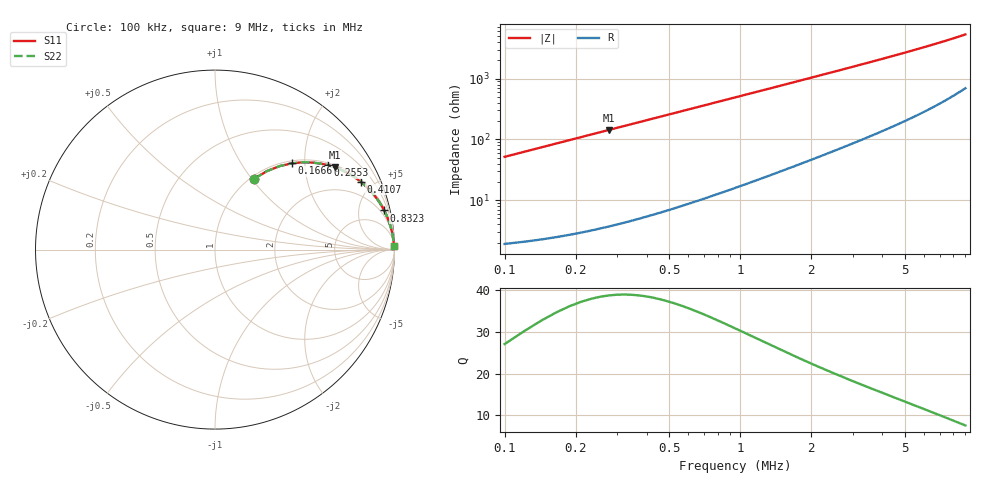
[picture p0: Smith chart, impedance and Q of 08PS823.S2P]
! Coilcraft 0805PS-823 Power Chip Inductor
! 5 February 2003
# MHZ S MA R 50
!Freq  MagS11  AngS11  MagS21  AngS21  MagS12  AngS12  MagS22  AngS22
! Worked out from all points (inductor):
!   403 points, 100 kHz to 9 MHz, reference 50 ohm
!   read as one part in series: L = 82 uH near 144.4 kHz
!   highest Q = 38.8 at 277.5 kHz (marker M1), where L = 82 uH
!   S11 on the Smith chart (normalised r, x): 100 kHz: 1.04, +1.03; 166.6 kHz: 1.05, +1.72; 255.3 kHz: 1.07, +2.63; 410.7 kHz: 1.11, +4.23; 832.3 kHz: 1.26, +8.58; 9 MHz: open
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0.1  0.4515 61.1  0.8758 -26.8  0.8758 -26.8  0.4515 61.1
0.12219  0.5252 56.5  0.8339 -31.7  0.8339 -31.7  0.5252 56.5
0.16657  0.6423 48.4  0.7482 -39.9  0.7482 -39.9  0.6423 48.4
0.21095  0.7263 41.9  0.6681 -46.6  0.6681 -46.6  0.7263 41.9
0.25533  0.7864 36.7  0.5977 -51.8  0.5977 -51.8  0.7864 36.7
0.27752  0.8098 34.5  0.5662 -54.0  0.5662 -54.0  0.8098 34.5
0.34409  0.8616 29.1  0.4859 -59.5  0.4859 -59.5  0.8616 29.1
0.41066  0.8952 25.0  0.423 -63.5  0.423 -63.5  0.8952 25.0
0.49942  0.9238 21.0  0.3589 -67.4  0.3589 -67.4  0.9238 21.0
0.58818  0.9419 18.1  0.3107 -70.3  0.3107 -70.3  0.9419 18.1
0.69913  0.9564 15.4  0.2654 -72.9  0.2654 -72.9  0.9564 15.4
0.83227  0.9673 13.0  0.2254 -75.2  0.2254 -75.2  0.9673 13.0
1.16512  0.9809 9.4  0.1631 -78.6  0.1631 -78.6  0.9809 9.4
1.58673  0.9879 6.9  0.1204 -80.8  0.1204 -80.8  0.9879 6.9
1.89739  0.9905 5.8  0.1008 -81.7  0.1008 -81.7  0.9905 5.8
2.25243  0.9924 4.9  0.08484 -82.4  0.08484 -82.4  0.9924 4.9
3.07346  0.9947 3.5  0.06187 -83.3  0.06187 -83.3  0.9947 3.5
3.76135  0.9956 2.9  0.0502 -83.6  0.0502 -83.6  0.9956 2.9
4.56019  0.9963 2.3  0.04097 -83.6  0.04097 -83.6  0.9963 2.3
6.04692  0.9969 1.7  0.03009 -83.3  0.03009 -83.3  0.9969 1.7
7.53365  0.9973 1.3  0.02332 -82.6  0.02332 -82.6  0.9973 1.3
9  0.9974 1.1  0.0187 -81.4  0.0187 -81.4  0.9974 1.1
